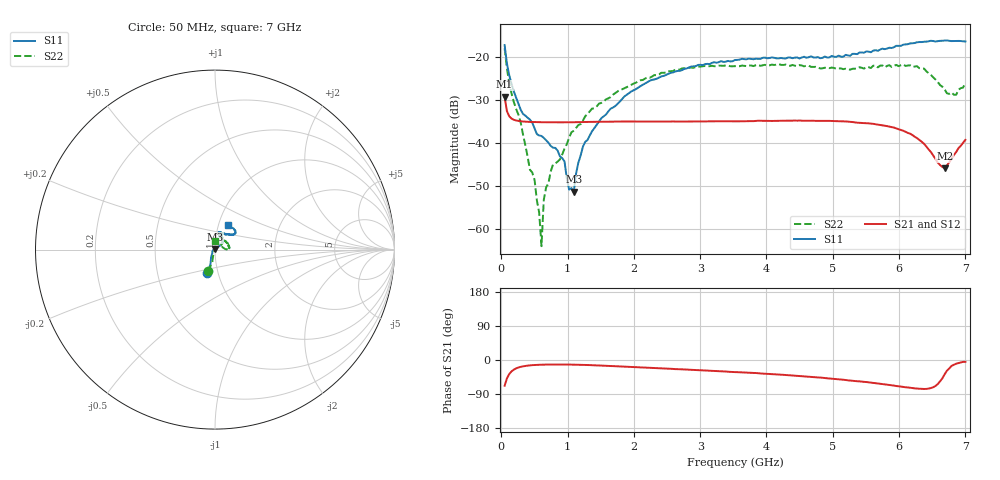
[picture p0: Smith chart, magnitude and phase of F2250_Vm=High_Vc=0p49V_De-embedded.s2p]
! Integrated Device Technology
! Corporate Headquarters
! 6024 Silver Creek Valley Road
! San Jose, CA 95138  USA
! Phone:  1-408-284-8200
! Toll Free:  1-800-223-1366
! Webpage:  http://www.idt.com/
! Timing and RF Division
! 515 Groton Road, Suite 102
! Westford, MA 01886-6024
! Device:  F2250
! Description: Voltage Variable RF Attenuator
! Frequency:  50.0 -  6000.00 MHz
! Package:  3x3 mm Thin QFN Plastic Package: 16 pin
! Ports:  2 RF, 3 DC
!  Pin  1  = GND
!  Pin  2  = NC
!  Pin  3  = RF1  = Port 1
!  Pin  4  = NC
!  Pin  5  = GND
!  Pin  6  = GND
!  Pin  7  = GND
!  Pin  8  = GND
!  Pin  9  = NC
!  Pin 10  = RF2  = Port 2
!  Pin 11  = NC
!  Pin 12  = GND
!  Pin 13  = GND
!  Pin 14  = VCNTRL
!  Pin 15  = VDD
!  Pin 16  = VMODE
! Vcntrl:  0.490 Volts
! Vmode:  +3.300 Volts
! Vdd:  +3.30  Volts
! Current:  1.267 mA
! Data:  The device was measured on a the F2250 evaluation board which has
!  individual transmission lines to the RF pins.  Data was collected
!  using a calibrated network analyzer.  The evaluation board was
!  de-embedded using a TRL calibration technique.
!  The reference plane is the edge of the package pin.
! Misc:  SN 10
!  Action Tracker AT0258
! Date Measured:  2014-11-26
! Date:  2015-10-15  MJV
! Note:
!  Integrated Device Technology supplies this data as a sample of measured
!  data at the package pin for this product.  Your particular data for this
!  product may vary.
!  Data was taken at 25 degrees C.
!  Integrated Device Technology reserves the right to change this data at anytime.
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# GHz S dB R 50
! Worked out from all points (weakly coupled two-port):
!   201 points, 50 MHz to 7 GHz, reference 50 ohm
!   highest |S21| = -29.23 dB at 50 MHz (marker M1); lowest = -45.9 dB at 6.687 GHz (marker M2)
!   lowest |S11| = -51.4 dB at 1.093 GHz (marker M3), VSWR 1.01, Z = 50 + j0.27 ohm
!   |S11| at or under -10 dB: start of sweep to end of sweep
!   |S22| runs from -64.1 to -17.9 dB; largest |S21 - S12| = 5.8e-05
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0.05  -17.17 -108.4  -29.23 -67.9  -29.23 -67.8  -17.91 -107.8
0.08475  -21.47 -107.4  -32.58 -48.6  -32.58 -48.6  -22.61 -102.3
0.189  -28.00 -119.9  -34.60 -25.4  -34.60 -25.4  -30.45 -107.4
0.50175  -36.63 -147.8  -35.13 -13.2  -35.13 -13.2  -48.61 -132.0
0.57125  -38.26 -161.0  -35.15 -12.6  -35.16 -12.6  -56.23 -168.4
0.606  -38.37 -162.4  -35.17 -12.4  -35.17 -12.4  -64.08 125.4
0.64075  -38.83 -162.4  -35.17 -12.2  -35.17 -12.2  -53.30 68.1
0.6755  -39.37 -163.8  -35.18 -12.1  -35.18 -12.1  -50.38 71.4
0.77975  -41.11 176.3  -35.19 -11.9  -35.19 -11.9  -45.05 70.3
0.9535  -44.31 170.8  -35.19 -12.0  -35.19 -12.0  -41.35 61.9
1.023  -50.89 140.4  -35.19 -12.1  -35.19 -12.2  -38.77 52.0
1.0925  -51.38 88.1  -35.17 -12.3  -35.17 -12.3  -37.14 50.1
1.2315  -40.84 40.3  -35.13 -12.8  -35.12 -12.8  -34.79 38.2
1.6485  -32.02 41.0  -35.05 -15.7  -35.05 -15.7  -29.31 40.2
2.37825  -24.75 46.6  -35.03 -21.8  -35.03 -21.8  -24.05 43.5
3.525  -20.66 71.7  -34.96 -31.7  -34.96 -31.7  -22.09 67.2
4.7065  -20.07 71.9  -34.82 -45.2  -34.83 -45.1  -22.28 66.9
5.85325  -17.79 40.5  -36.21 -65.9  -36.21 -66.0  -21.87 17.9
6.3745  -16.40 40.9  -40.18 -76.5  -40.18 -76.6  -22.64 1.5
6.68725  -16.12 47.8  -45.88 -37.7  -45.87 -37.5  -27.52 23.6
6.861  -16.22 54.5  -42.12 -9.7  -42.07 -9.8  -28.77 58.6
7  -16.33 62.4  -39.27 -4.8  -39.24 -5.0  -25.93 88.4
